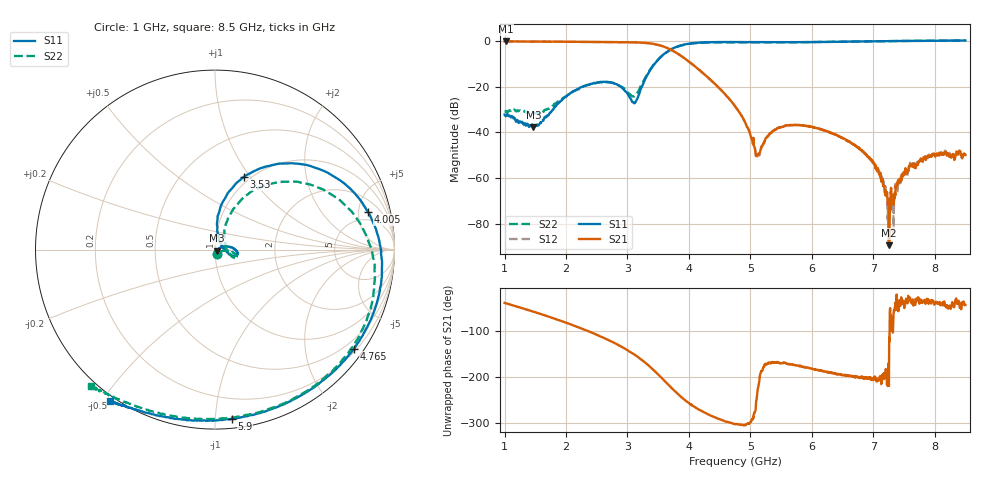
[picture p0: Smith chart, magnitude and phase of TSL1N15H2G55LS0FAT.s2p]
!TSL1N15H2G55LS0FAT  S-PARAMETER MODEL  ( General Type )
! Model Generated by TAIYO YUDEN Corporation (https://www.yuden.co.jp/en/)
! Version 1.0
! TAIYO YUDEN Control No. 240527
! Copyright(c) 2024 TAIYO YUDEN CO.,LTD. All Rights Reserved.
! Products Name : Ceramic RF Devices
! Characteristics :
!  Passband freq :1710-2700MHz, , ( At Passband , Insertion Loss :0.7dB, VSWR 2.0 )
!  Attenuation :22 dB min at 4600to 5400MHz,25 dB min at 4800to 8100MHz, Impedance : 50 Ohm
!  Case Size : 1 x 0.5 / 0.039 x 0.02 [mm/inch] , Thickness : 0.4 / 0.016 [mm/inch]
!  (Conditions: Temperature = 25 degC , DC Bias Current/Voltage = 0A / 0V)
! External Node Assignments :
!  1  o---|-------|---o  2
!  |  LPF  |
! GND o---|-------|---o GND
! Frequency Range : 1GHz  -  8.5GHz  [ 1501 STEP ]
# MHz S RI R 50
! Freq[MHz].  S11 Real  S11 Imag  S21 Real  S21 Imag  S12 Real  S12 Imag  S22 Real  S22 Imag
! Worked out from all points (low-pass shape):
!   1501 points, 1 GHz to 8.5 GHz, reference 50 ohm
!   highest |S21| = -0.13 dB at 1.015 GHz (marker M1); lowest = -89.4 dB at 7.26 GHz (marker M2)
!   |S21| within 3 dB of the highest: start of sweep to 3.655 GHz
!   lowest |S11| = -37.7 dB at 1.47 GHz (marker M3), VSWR 1.03, Z = 51.1 - j0.66 ohm
!   |S11| at or under -10 dB: start of sweep to 3.441 GHz
!   |S22| runs from -31.8 to 0.3 dB; largest |S21 - S12| = 0.0094
!   S11 on the Smith chart (normalised r, x): 1 GHz: 1.02, -0.05; 3.53 GHz: 0.93, +0.93; 4.005 GHz: 3.45, +6.36; 4.765 GHz: 0.27, -3.11; 5.9 GHz: 0.06, -1.10; 8.5 GHz: -0.02, -0.52
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1000  0.00899 -0.0229  0.7627 -0.6222  0.7615 -0.6228  0.0113 -0.0263
1015  0.00797 -0.0213  0.7579 -0.6286  0.7548 -0.6306  0.0115 -0.0254
1470  0.0114 -0.00645  0.5113 -0.8275  0.5133 -0.83  0.0174 -0.0195
2250  0.0971 0.00941  -0.0739 -0.9582  -0.0748 -0.959  0.0942 -0.014
2750  0.1167 -0.0348  -0.5223 -0.7908  -0.5238 -0.7917  0.1126 -0.0457
3110  0.0387 0.0212  -0.8166 -0.4569  -0.8176 -0.4574  0.0569 0.0224
3500  0.1238 0.375  -0.7967 0.2006  -0.7986 0.2001  0.2169 0.3315
3530  0.1589 0.4041  -0.7637 0.2486  -0.7639 0.2486  0.2563 0.3504
4005  0.8523 0.211  -0.0817 0.3407  -0.0821 0.3403  0.8679 0.0133
4750  0.7817 -0.5424  0.0197 0.0321  0.0196 0.0319  0.6277 -0.6975
4765  0.775 -0.5522  0.0183 0.0299  0.0181 0.0298  0.6192 -0.7065
5120  0.5804 -0.7453  -0.00227 0.00233  -0.00229 0.00228  0.3941 -0.8519
5395  0.4129 -0.8475  -0.011 -0.00218  -0.0112 -0.00221  0.219 -0.9123
5900  0.0938 -0.9423  -0.0139 -0.000172  -0.0141 -0.000222  -0.0826 -0.9426
6000  0.0339 -0.9494  -0.0133 0.000341  -0.0131 0.000494  -0.1376 -0.9405
6865  -0.3535 -0.9158  -0.00309 0.00128  -0.0033 0.00135  -0.4719 -0.8599
7135  -0.429 -0.8952  -0.000694 0.000439  -0.00104 0.000417  -0.5337 -0.8339
7250  -0.4506 -0.8892  -0.000252 -4.52e-05  -2.85e-05 -1.52e-05  -0.5536 -0.8293
7260  -0.4537 -0.8876  -1.38e-05 -3.08e-05  -0.000129 -5.26e-05  -0.5555 -0.8284
7385  -0.4781 -0.8803  0.0005 -0.000446  0.000452 -0.00052  -0.5832 -0.8133
7625  -0.5128 -0.8686  0.00153 -0.00129  0.00155 -0.00131  -0.614 -0.8021
8500  -0.5865 -0.8434  0.0023 -0.00219  0.0025 -0.00232  -0.6924 -0.7612
